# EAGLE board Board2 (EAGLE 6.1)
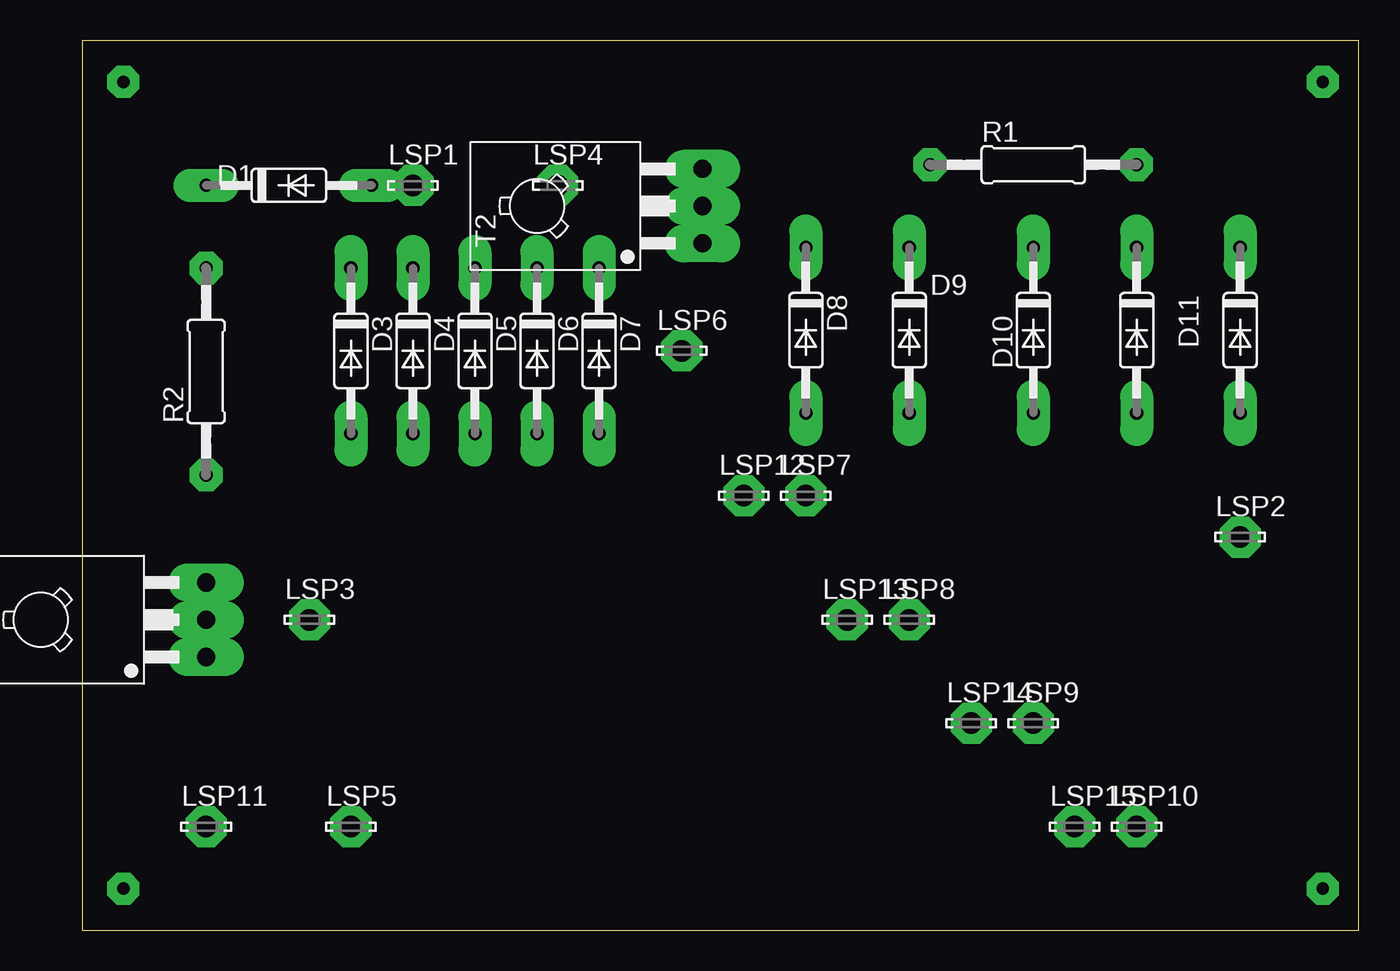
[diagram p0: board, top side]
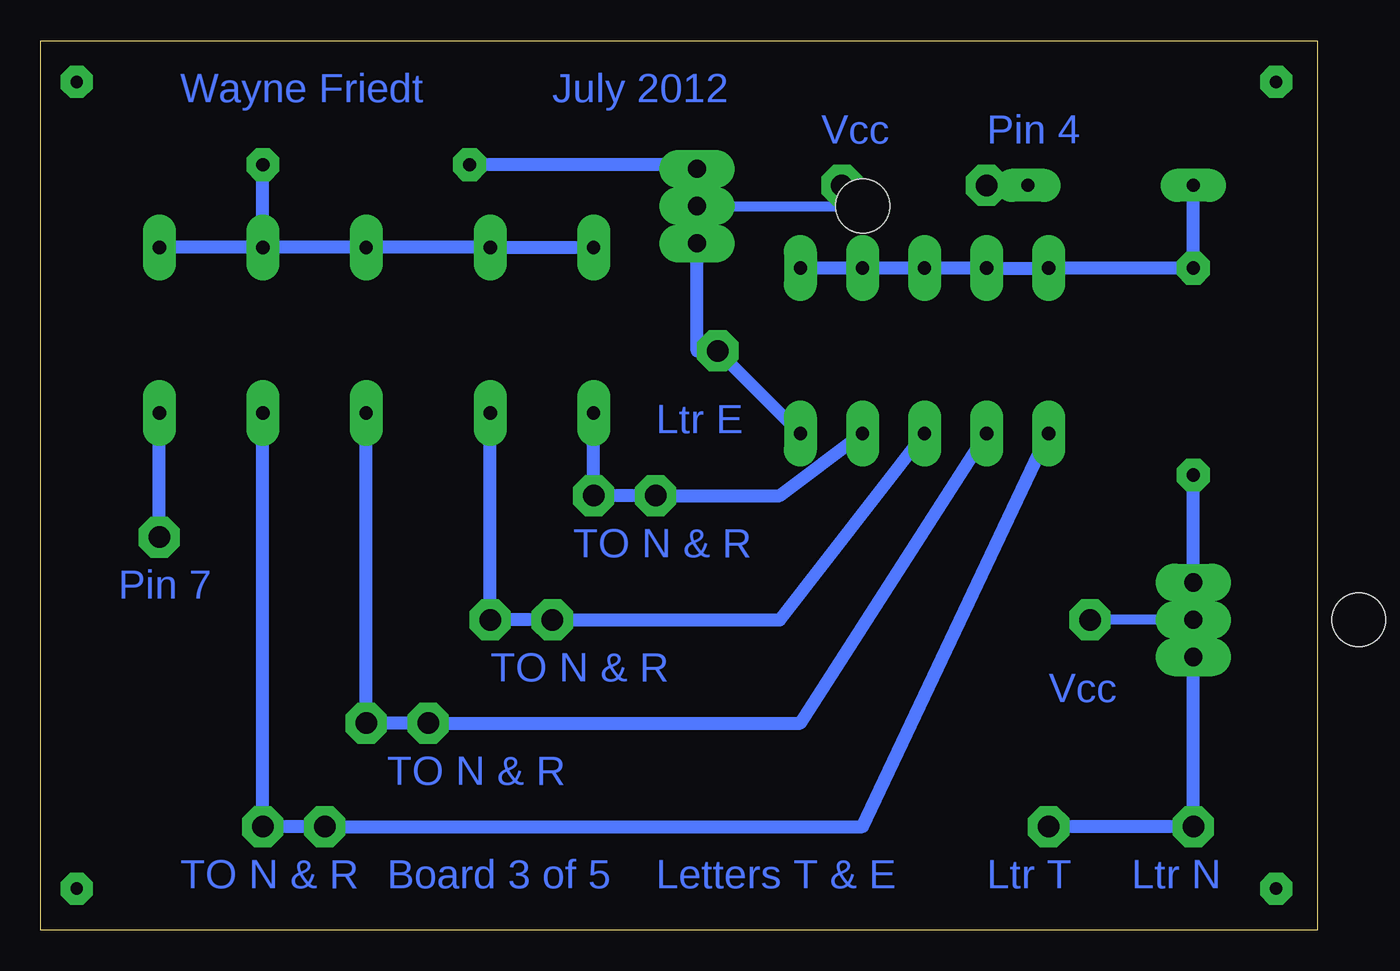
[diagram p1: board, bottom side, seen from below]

Size 78.41 x 54.6 mm. Coordinates in mm from the lower left corner, seen from the top.
Outline: 0,0 78.41,0 78.41,54.6 0,54.6 0,0
Copper layers (1*16): Top 0.035mm / dielectric 1.5mm / Bottom 0.035mm
Design rules: minimum track width 0.8mm, minimum drill 0.8mm, track to track 0.8mm, track to pad 0.8mm, pad to pad 0.45mm, via to via 0.8mm, smd to smd 8mil, copper to edge 10mil, drill to drill 8mil, minimum pad ring 0.6mm, minimum via ring 0.6mm, stop-mask expansion 0mil, vias tented up to drill 0mil, thermal gap 10mil

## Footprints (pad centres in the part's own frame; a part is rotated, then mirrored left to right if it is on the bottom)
DO35-10 = drill 0.813 long: A 5.08,0; C -5.08,0
LSP13 = drill 1.321 pad 2.159 octagon: MP 0,0
0207/12 = drill 0.813 octagon: 1 -6.35,0; 2 6.35,0
TO126 = drill 1.118 long: 1 -2.286,-5.08; 2 0,-5.08; 3 2.286,-5.08 | hole 3.302: 0,5.08

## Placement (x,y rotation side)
D1  1N4148DO35-10  [DO35-10]  12.7,45.72 0 top
D2  1N4148DO35-10  [DO35-10]  71.12,36.83 270 top
D3  1N4148DO35-10  [DO35-10]  16.51,35.56 270 top
D4  1N4148DO35-10  [DO35-10]  20.32,35.56 270 top
D5  1N4148DO35-10  [DO35-10]  24.13,35.56 270 top
D6  1N4148DO35-10  [DO35-10]  27.94,35.56 270 top
D7  1N4148DO35-10  [DO35-10]  31.75,35.56 270 top
D8  1N4148DO35-10  [DO35-10]  44.45,36.83 270 top
D9  1N4148DO35-10  [DO35-10]  50.8,36.83 270 top
D10  1N4148DO35-10  [DO35-10]  58.42,36.83 270 top
D11  1N4148DO35-10  [DO35-10]  64.77,36.83 270 top
LSP1  LSP13  [LSP13]  20.32,45.72 0 top
LSP2  LSP13  [LSP13]  71.12,24.13 0 top
LSP3  LSP13  [LSP13]  13.97,19.05 0 top
LSP4  LSP13  [LSP13]  29.21,45.72 0 top
LSP5  LSP13  [LSP13]  16.51,6.35 0 top
LSP6  LSP13  [LSP13]  36.83,35.56 0 top
LSP7  LSP13  [LSP13]  44.45,26.67 0 top
LSP8  LSP13  [LSP13]  50.8,19.05 0 top
LSP9  LSP13  [LSP13]  58.42,12.7 0 top
LSP10  LSP13  [LSP13]  64.77,6.35 0 top
LSP11  LSP13  [LSP13]  7.62,6.35 0 top
LSP12  LSP13  [LSP13]  40.64,26.67 0 top
LSP13  LSP13  [LSP13]  46.99,19.05 0 top
LSP14  LSP13  [LSP13]  54.61,12.7 0 top
LSP15  LSP13  [LSP13]  60.96,6.35 0 top
R1  330R  [0207/12]  58.42,46.99 0 top
R2  330R  [0207/12]  7.62,34.29 90 top
T1  BD139  [TO126]  2.54,19.05 90 top
T2  BD139  [TO126]  33.02,44.45 90 top

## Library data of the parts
D1-D11 = diode
LSP1-LSP15 = solpad
R1 R2 = resistor
T1 T2 = transistor

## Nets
N$1: LSP5.MP LSP11.MP T1.1
N$2: LSP3.MP T1.2
N$3: R2.1 T1.3
N$4: D1.C D3.C D4.C D5.C D6.C D7.C R2.2
N$5: D7.A LSP6.MP T2.1
N$6: LSP4.MP T2.2
N$7: R1.1 T2.3
N$8: D2.C D8.C D9.C D10.C D11.C R1.2
N$9: D2.A LSP2.MP
N$10: D6.A D8.A LSP7.MP LSP12.MP
N$11: D5.A D9.A LSP8.MP LSP13.MP
N$12: D4.A D10.A LSP9.MP LSP14.MP
N$13: D3.A D11.A LSP10.MP LSP15.MP
N$14: D1.A LSP1.MP

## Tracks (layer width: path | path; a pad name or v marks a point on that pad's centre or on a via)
N$1
  Bottom 0.8: T1.1 LSP11.MP LSP5.MP
N$2
  Bottom 0.61: T1.2 LSP3.MP
N$3
  Bottom 0.8: T1.3 R2.1
N$4
  Bottom 0.8: D7.C D6.C D5.C D4.C D3.C R2.2 D1.C
N$5
  Bottom 0.8: D7.A LSP6.MP 38.1,35.56 T2.1
N$6
  Bottom 0.61: T2.2 29.21,44.45 LSP4.MP
N$7
  Bottom 0.8: R1.1 38.1,46.99 T2.3
N$8
  Bottom 0.8: D8.C D9.C D10.C D11.C | D11.C R1.2 | D11.C D2.C
N$9
  Bottom 0.8: LSP2.MP D2.A
N$10
  Bottom 0.8: D8.A LSP7.MP LSP12.MP 33.02,26.67 D6.A
N$11
  Bottom 0.8: D9.A LSP8.MP LSP13.MP 33.02,19.05 D5.A
N$12
  Bottom 0.8: D10.A LSP9.MP LSP14.MP 31.75,12.7 D4.A
N$13
  Bottom 0.8: D11.A LSP10.MP LSP15.MP 27.94,6.35 D3.A
N$14
  Bottom 0.8: LSP1.MP D1.A
S$1  (via drill 0.76)
  other vias: 2.54,52.07 76.2,52.07 76.2,2.54 2.54,2.54

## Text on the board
Bottom: July 2012 | Wayne Friedt | Pin 4 | Vcc | Ltr E | TO N & R | Pin 7 | TO N & R | Vcc | TO N & R | Ltr N | Ltr T | Letters T & E | Board 3 of 5 | TO N & R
